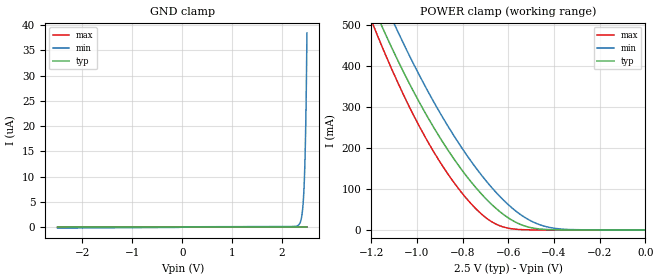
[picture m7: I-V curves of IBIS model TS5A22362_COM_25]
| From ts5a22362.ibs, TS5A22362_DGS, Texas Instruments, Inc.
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[Model]   TS5A22362_COM_25
Model_type  Terminator
| variable   typ   min   max
C_comp   147.54pF   113.80pF   178.96pF
| C_tri-state   147.54pF   113.80pF   178.96pF
[Temperature Range]   40   100   -40
| Ambient temperature   25   85   -40
[Voltage range]   2.5   2.3   2.7
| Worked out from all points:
|   POWER clamp passes 1 mA (typ) near -0.43 V on its own axis
[GND Clamp]
| TS5A22362_COM_25
|   Voltage   I(typ)   I(min)   I(max)
-2.5V     -5.094nA   -230.8nA   -2.936nA
2.325V    3.069nA    333.2nA    2.348nA
2.365V    3.124nA    903.5nA    2.391nA
2.395V    3.171nA    2.078uA    2.423nA
2.42V     3.225nA    4.218uA    2.45nA
2.44V     3.29nA     7.417uA    2.471nA
2.45V     3.338nA    9.815uA    2.482nA
2.46V     3.403nA    12.96uA    2.493nA
2.475V    3.55nA     19.59uA    2.509nA
2.485V    3.7nA      25.71uA    2.52nA
2.49V     3.798nA    29.43uA    2.525nA
2.5V      4.058nA    38.47uA    2.536nA
[POWER Clamp]
| TS5A22362_COM_25
|   Voltage   I(typ)   I(min)   I(max)
-2.5V     3.153A     3.212A     3.436A
-1.19V    544.3mA    618.4mA    499.2mA
-1.175V   525.1mA    598.8mA    478.5mA
-1.14V    481.4mA    553.9mA    431.5mA
-1.08V    410.2mA    480.5mA    355.8mA
-955mV    277.7mA    341.9mA    218.4mA
-805mV    147.9mA    201.9mA    91.82mA
-690mV    71.83mA    115.1mA    26.57mA
-570mV    19.59mA    47.49mA    1.921mA
-480mV    3.571mA    16.62mA    107.3uA
-395mV    431.3uA    3.815mA    4.236uA
0V        0A         0A         0A
